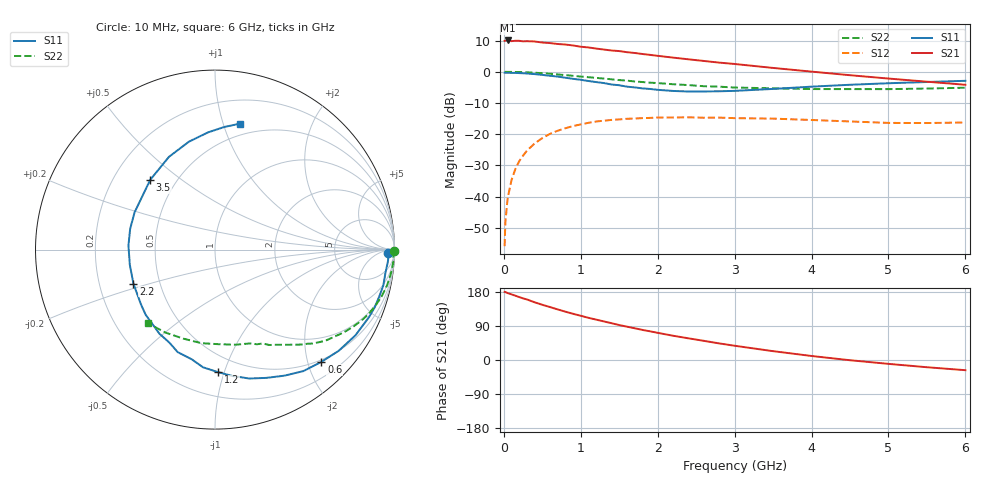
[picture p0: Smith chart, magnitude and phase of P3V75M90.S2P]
! SIEMENS Small Signal Semiconductors
! BFP181
! Si NPN RF Bipolar Junction Transistor in SOT143
! VCE = 0.75 V  IC = 0.9 mA
! Common Emitter S-Parameters:  March  1996
# GHz  S  MA  R  50
!  f  S11  S21  S12  S22
! GHz  MAG  ANG  MAG  ANG  MAG  ANG  MAG  ANG
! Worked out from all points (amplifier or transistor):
!   36 points, 10 MHz to 6 GHz, reference 50 ohm
!   highest |S21| = 10.0 dB at 50 MHz (marker M1)
!   |S21| within 3 dB of that: start of sweep to 1.33 GHz
!   unconditionally stable (mu >= 1): 2.925 GHz to end of sweep
!   at 250 MHz: K = 0.09, MSG = 18.3 dB, |S12| = -26.9 dB
!   at 1.4 GHz: K = 0.53, MSG = 11.1 dB, |S12| = -15.4 dB
!   at 6 GHz: K = 1.44, MAG = 2.1 dB, |S12| = -16.3 dB
!   S11 on the Smith chart (normalised r, x): 10 MHz: 45, -22; 600 MHz: 0.46, -2.25; 1.2 GHz: 0.37, -0.95; 2.2 GHz: 0.35, -0.18; 3.5 GHz: 0.36, +0.39; 6 GHz: 0.40, +1.14
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0.01  0.9649 -1.0  3.123 179.7  0.0016 90.4  0.9973 -0.3
0.02  0.9669 -1.7  3.151 179.3  0.0039 87.0  0.9965 -0.8
0.05  0.9661 -3.7  3.174 176.6  0.0095 90.3  0.9948 -2.0
0.1  0.9583 -8.0  3.096 173.2  0.0184 84.2  0.9955 -4.0
0.2  0.9518 -15.9  3.131 166.0  0.0369 79.3  0.9884 -8.0
0.4  0.9168 -31.4  3.057 152.3  0.0709 69.0  0.965 -15.6
0.6  0.8619 -46.5  2.881 139.7  0.101 59.0  0.9285 -22.7
0.8  0.8016 -61.2  2.731 127.5  0.1244 50.1  0.8835 -28.9
0.9  0.7698 -68.2  2.637 121.9  0.1348 45.9  0.8602 -31.8
1.1  0.7105 -82.2  2.452 111.3  0.1518 38.4  0.8171 -36.9
1.2  0.6832 -88.5  2.353 106.6  0.1593 34.7  0.7977 -39.5
1.5  0.6078 -110.0  2.145 92.2  0.1722 25.9  0.7352 -45.5
1.7  0.5616 -123.5  2 83.8  0.1779 20.8  0.6991 -49.3
2  0.5131 -143.5  1.8 71.7  0.1846 14.5  0.6581 -53.7
2.2  0.4924 -157.4  1.685 64.0  0.1848 10.3  0.6308 -57.2
2.8  0.4866 166.3  1.401 43.8  0.184 0.9  0.5766 -66.2
3  0.4938 155.2  1.332 37.6  0.1804 -1.9  0.5583 -69.4
3.5  0.5304 132.9  1.151 23.3  0.1773 -6.4  0.5424 -77.6
4  0.577 116.4  1.005 10.6  0.1685 -10.2  0.5278 -87.4
4.5  0.6185 103.6  0.88 -0.6  0.1598 -13.1  0.5269 -98.3
5.5  0.6849 85.7  0.693 -19.1  0.1506 -10.8  0.5383 -120.7
6  0.7159 78.7  0.618 -26.9  0.1538 -9.7  0.5547 -132.1
